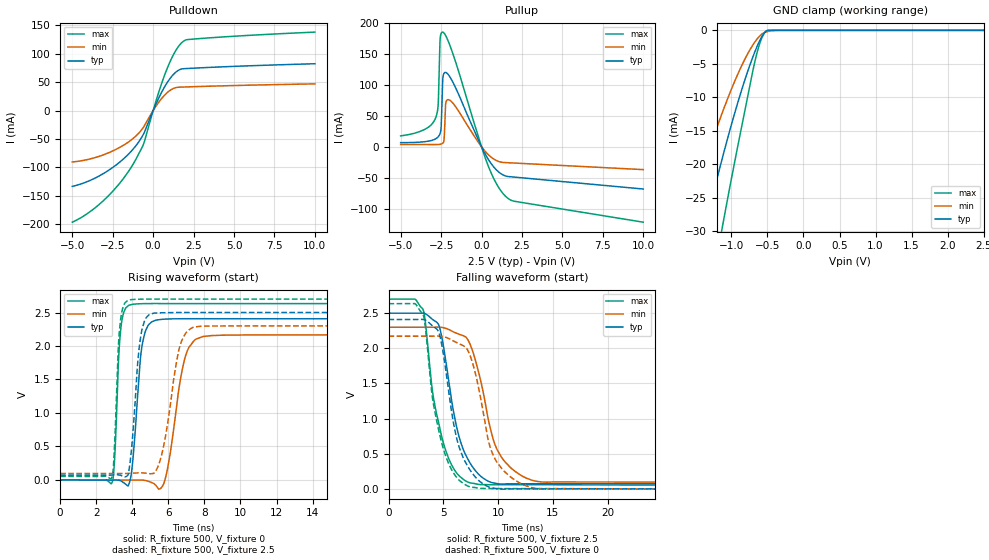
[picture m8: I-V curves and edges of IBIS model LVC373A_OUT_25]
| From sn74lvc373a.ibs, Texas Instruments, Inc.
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[Model]   LVC373A_OUT_25
Model_type  3-state
Enable   Active-Low
Vref =   0
Rref =   500
Cref =   30p
Vmeas =   1.25
| variable   typ   min   max
C_comp   3.25pF   2.90pF   3.70pF
| C_pullup   6.10pF   3.10pF   9.05pF
| C_pulldown   6.16pF   3.02pF   9.44pF
| C_tri-state   3.25pF   2.90pF   3.70pF
[Temperature Range]   40   100   -40
| Ambient temperature   25   85   -40
[Voltage range]   2.5   2.3   2.7
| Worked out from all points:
|   slope of the pulldown table from 0 to 0.375 V, typ, clamps not added: 15.7 ohm
|   slope of the pullup table from 0 to 0.375 V, typ, clamps not added: 20.3 ohm
|   GND clamp passes 1 mA (typ) near -0.58 V on its own axis
|   rising waveform, R_fixture 500, V_fixture 0: 20-80 % time 409ps typ, 718ps min, 252ps max; typ from 0 V to 2.41 V
|   falling waveform, R_fixture 500, V_fixture 2.5: 20-80 % time 1.8ns typ, 2.11ns min, 1.64ns max; typ from 2.5 V to 0.072 V
|   rising waveform, R_fixture 500, V_fixture 2.5: 20-80 % time 413ps typ, 758ps min, 242ps max; typ from 0.072 V to 2.5 V
|   falling waveform, R_fixture 500, V_fixture 0: 20-80 % time 1.72ns typ, 1.93ns min, 1.6ns max; typ from 2.41 V to 0 V
[GND Clamp]
| LVC373A_OUT_25
|   Voltage   I(typ)   I(min)   I(max)
-5V       -227.5mA   -167.1mA   -315.1mA
-1.675V   -43.93mA   -30.24mA   -64.16mA
-1.62V    -41.29mA   -28.31mA   -60.51mA
-1.35V    -28.79mA   -19.21mA   -43.1mA
-1.155V   -20.36mA   -13.18mA   -31.21mA
-1.11V    -18.51mA   -11.88mA   -28.56mA
-860mV    -9.029mA   -5.369mA   -14.59mA
-660mV    -2.848mA   -1.541mA   -4.058mA
-590mV    -1.19mA    -686uA     -1.49mA
-520mV    -140.4uA   -252.6uA   -137.6uA
-315mV    -52.46nA   -1.806uA   -6.57nA
2.5V      16.74pA    19.24nA    6.67pA
[Pulldown]
| LVC373A_OUT_25
|   Voltage   I(typ)   I(min)   I(max)
-5V       -133.4mA   -90.34mA   -196.5mA
-4.005V   -124.2mA   -85.84mA   -180.1mA
-3.005V   -109.6mA   -77.11mA   -156.7mA
-2.07V    -90.78mA   -64.86mA   -127.9mA
-1.285V   -69.31mA   -50.1mA    -96.5mA
-580mV    -40.39mA   -28.39mA   -57.82mA
275mV     17.84mA    11.98mA    26.11mA
890mV     50.28mA    32.17mA    75.77mA
1.385V    67.28mA    40.38mA    105.1mA
1.845V    73.75mA    41.51mA    121.5mA
3.38V     76mA       42.93mA    128mA
10V       82.59mA    47.12mA    138.3mA
[Pullup]
| LVC373A_OUT_25
|   Voltage   I(typ)   I(min)   I(max)
-5V       6.743mA    3.718mA    17.64mA
-2.84V    12.84mA    3.59mA     46.48mA
-2.685V   16mA       3.703mA    66.76mA
-2.565V   21.31mA    4.055mA    172.1mA
-2.51V    27.95mA    4.376mA    182.6mA
-2.39V    111.6mA    6.017mA    185.6mA
-2.315V   119.1mA    11.8mA     184mA
-2.215V   120.3mA    70mA       179.9mA
-2.02V    115.7mA    76.16mA    168.5mA
305mV     -15.36mA   -9.722mA   -23.43mA
1.495V    -47.3mA    -25.59mA   -80.4mA
10V       -68.37mA   -36.95mA   -122.1mA
[Ramp]
| LVC373A_OUT_25
| variable   typ   min   max
dV/dt_r   1.50/4.49E-10   1.38/7.82E-10   1.61/2.69E-10
dV/dt_f   1.46/1.85E-09   1.32/2.16E-09   1.59/1.66E-09
R_load = 500
[Rising Waveform]
| LVC373A_OUT_25
R_fixture =   500
C_fixture =   0
L_fixture =   0
V_fixture =   0
V_fixture_min = 0
V_fixture_max = 0
|   Time   V(typ)   V(min)   V(max)
0s        181.1pV    4.724nV    128.7pV
2.89ns    -1.276mV   110.7uV    -33.11mV
3.375ns   -14.63mV   -1.384mV   2.286V
4.01ns    237.3mV    -924.4uV   2.622V
4.55ns    2.018V     -978.2uV   2.632V
5.38ns    2.389V     -104.1mV   2.634V
5.905ns   2.401V     102.3mV    2.633V
6.96ns    2.407V     1.857V     2.633V
7.93ns    2.407V     2.142V     2.633V
50ns      2.406V     2.166V     2.633V
[Falling Waveform]
| LVC373A_OUT_25
R_fixture =   500
C_fixture =   0
L_fixture =   0
V_fixture =   2.5
V_fixture_min = 2.3
V_fixture_max = 2.7
|   Time   V(typ)   V(min)   V(max)
0s        2.5V       2.3V       2.7V
3.145ns   2.501V     2.3V       2.556V
4.015ns   2.412V     2.3V       1.388V
4.57ns    2.338V     2.301V     944.3mV
5.325ns   1.723V     2.279V     500.5mV
6.205ns   891.2mV    2.215V     228.2mV
7.355ns   391.3mV    2.09V      89.39mV
9.865ns   75.93mV    575.1mV    57.67mV
13.1ns    71.88mV    122.5mV    57.72mV
50ns      72.12mV    96.87mV    53.92mV
[Rising Waveform]
| LVC373A_OUT_25
R_fixture =   500
C_fixture =   0
L_fixture =   0
V_fixture =   2.5
V_fixture_min = 2.3
V_fixture_max = 2.7
|   Time   V(typ)   V(min)   V(max)
0s        72.03mV    96.79mV    53.9mV
2.85ns    72.45mV    96.81mV    28.71mV
2.985ns   74.73mV    96.7mV     342.5mV
3.3ns     73.36mV    95.99mV    2.264V
3.92ns    361.2mV    99.35mV    2.691V
4.475ns   2.153V     106.3mV    2.699V
5.19ns    2.49V      98.28mV    2.701V
6.63ns    2.5V       1.988V     2.7V
7.44ns    2.5V       2.283V     2.7V
50ns      2.5V       2.3V       2.7V
[Falling Waveform]
| LVC373A_OUT_25
R_fixture =   500
C_fixture =   0
L_fixture =   0
V_fixture =   0
V_fixture_min = 0
V_fixture_max = 0
|   Time   V(typ)   V(min)   V(max)
0s        2.41V      2.173V     2.635V
2.375ns   2.41V      2.173V     2.636V
3.145ns   2.411V     2.173V     2.487V
4ns       2.322V     2.173V     1.309V
4.57ns    2.238V     2.174V     844.2mV
6.15ns    768.6mV    2.087V     176.2mV
7.36ns    288.1mV    1.931V     32.56mV
9.49ns    11.11mV    505.1mV    3.617mV
12.88ns   -91.4uV    25.05mV    3.762mV
50ns      82.63uV    80.69uV    18.68uV
